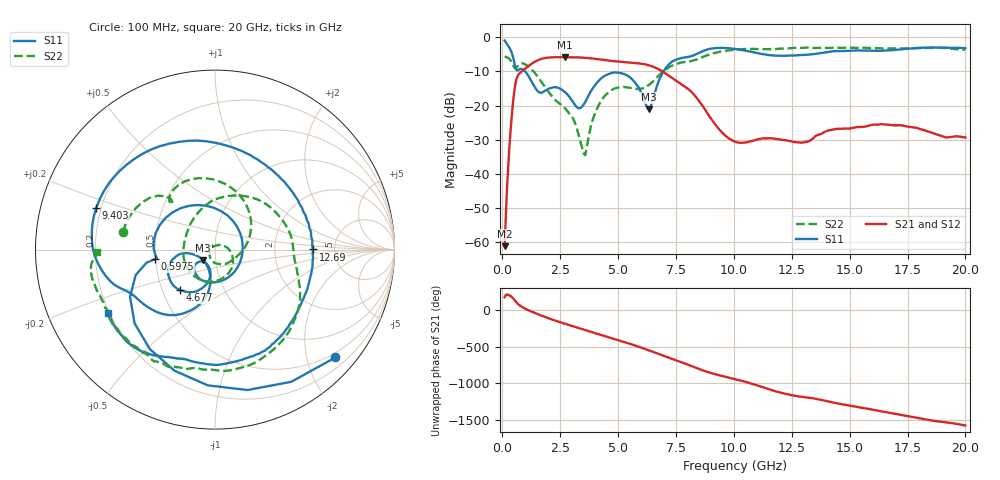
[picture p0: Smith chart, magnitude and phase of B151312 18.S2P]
!  2-Port S-parameters saved by WinCal
! VAR MeasName=S-Parameters (CALIBRATED_DATA) read from VNA (N5244A)
! VAR MeasDate=12/8/2015 5:44:53 PM
! VAR NAME=B151312 18
! VAR FILENAME=B151312 18.S2P
! VAR DATE=12/8/2015 5:44:53 PM
! VAR PHYS_PORTS=1,2
# Hz S DB R 50
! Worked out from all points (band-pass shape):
!   401 points, 100 MHz to 20 GHz, reference 50 ohm
!   highest |S21| = -5.82 dB at 2.687 GHz (marker M1); lowest = -61.2 dB at 100 MHz (marker M2)
!   |S21| within 3 dB of the highest: 1.056 GHz to 6.584 GHz (5.529 GHz wide, 145 % of centre)
!   lowest |S11| = -21.1 dB at 6.319 GHz (marker M3), VSWR 1.19, Z = 43.5 - j5.15 ohm
!   |S11| at or under -10 dB: 987.5 MHz to 6.959 GHz (5.972 GHz wide, 150 % of centre)
!   |S22| runs from -34.6 to -3.0 dB; largest |S21 - S12| = 0.0015
!   S11 on the Smith chart (normalised r, x): 100 MHz: 0.40, -2.56; 597.5 MHz: 0.50, -0.06; 4.677 GHz: 0.62, -0.31; 9.403 GHz: 0.18, +0.17; 12.69 GHz: 3.40, +0.01; 20 GHz: 0.19, -0.27
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1e8  -0.91 -41.9  -61.21 177.4  -61.45 175.0  -5.64 169.3
3.4875e8  -3.58 -123.3  -28.16 -164.1  -28.14 -164.1  -6.65 141.8
5.975e8  -9.38 -170.8  -12.61 113.6  -12.61 113.5  -9.04 134.1
1.294e9  -13.28 81.0  -7.61 -22.2  -7.61 -22.2  -9.59 65.4
1.94075e9  -15.27 -65.9  -5.97 -103.4  -5.97 -103.4  -15.46 4.9
2.687e9  -15.93 -136.8  -5.82 177.0  -5.81 177.0  -20.64 -60.2
3.43325e9  -20.38 -114.8  -5.93 103.0  -5.93 102.9  -31.91 176.4
3.5825e9  -18.94 -104.5  -5.99 88.3  -5.99 88.3  -34.56 105.1
4.12975e9  -12.99 -108.2  -6.39 34.8  -6.38 34.7  -20.33 -14.3
4.677e9  -10.53 -130.7  -6.88 -17.8  -6.87 -17.8  -15.67 -74.9
5.473e9  -11.51 -162.5  -7.35 -95.7  -7.35 -95.9  -14.76 -153.1
6.31875e9  -21.06 -138.4  -8.16 172.1  -8.17 172.1  -13.98 132.3
6.7665e9  -12.62 -98.8  -9.40 119.5  -9.39 119.5  -11.15 90.6
7.61225e9  -6.29 -136.6  -13.15 23.2  -13.11 23.1  -7.59 19.0
9.40325e9  -3.08 160.6  -27.23 -172.8  -27.23 -173.3  -4.19 -48.7
1.005e10  -3.40 131.8  -30.56 136.9  -30.59 136.6  -3.59 -67.6
1.1244e10  -4.89 74.7  -29.61 25.3  -29.71 25.4  -3.49 -93.6
1.268675e10  -5.26 0.1  -30.75 -94.0  -30.77 -93.6  -3.08 -112.2
1.338325e10  -4.97 -30.8  -29.82 -124.2  -29.78 -123.7  -3.10 -121.5
1.4627e10  -4.01 -73.5  -26.80 155.0  -26.75 155.2  -3.09 -134.4
1.67165e10  -3.82 -110.8  -25.66 34.3  -25.51 34.4  -3.20 -152.2
2e10  -3.19 -149.2  -29.34 -137.5  -29.39 -138.7  -3.66 -179.0
